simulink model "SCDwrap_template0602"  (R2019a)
settings: configuration reference "configurationSettings" (kept in a data dictionary, not in this file)
undefined symbols (not defined in the file or in its folder): SCDnode06params

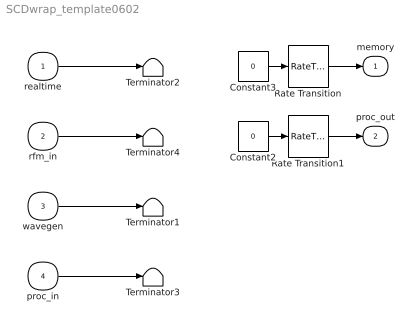
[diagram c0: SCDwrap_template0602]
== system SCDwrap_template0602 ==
  realtime : Inport  OutDataTypeStr=single  SampleTime=SCDnode06params.timing.thperiod(2)
  rfm_in : Inport  Port=2  OutDataTypeStr=Bus: RFMINbus  SampleTime=SCDnode06params.timing.thperiod(2)
  wavegen : Inport  Port=3  OutDataTypeStr=Bus: WG0602bus  SampleTime=SCDnode06params.timing.thperiod(2)
  proc_in : Inport  Port=4  OutDataTypeStr=Bus: PROCIN06bus  SampleTime=SCDnode06params.timing.thperiod(2)
  Constant2 : Constant  Value=0  OutDataTypeStr=Bus: PROCOUT0602bus
  Constant3 : Constant  Value=0  OutDataTypeStr=Bus: MEM0602bus
  Rate Transition : RateTransition
  Rate Transition1 : RateTransition
  Terminator{1..4} (4 alike) : Terminator
  memory : Outport  OutDataTypeStr=Bus: MEM0602bus  SampleTime=SCDnode06params.timing.thperiod(2)
  proc_out : Outport  Port=2  OutDataTypeStr=Bus: PROCOUT0602bus  SampleTime=SCDnode06params.timing.thperiod(2)
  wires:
  Constant2/1 -> Rate Transition1/1
  Constant3/1 -> Rate Transition/1
  rfm_in/1 -> Terminator4/1
  wavegen/1 -> Terminator1/1
  proc_in/1 -> Terminator3/1
  Rate Transition/1 -> memory/1
  Rate Transition1/1 -> proc_out/1
  realtime/1 -> Terminator2/1
